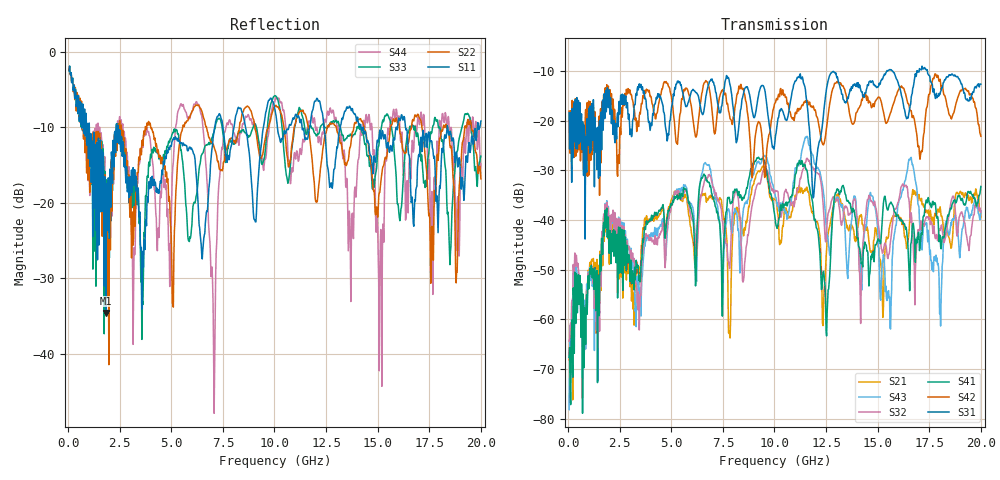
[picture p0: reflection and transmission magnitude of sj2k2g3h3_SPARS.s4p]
! FILE: E:\users\goganessyan\GBX_Backplane\FR408_backplane\1m_OUTBOUND_NEXT\sj2k2g3h3_SPARS.s4p
# MHZ S RI R 50.00
! FREQ  S11  S12  S13  S14
!  S21  S22  S23  S24
!  S31  S32  S33  S34
!  S41  S42  S43  S44
!  REAL  IMAG  REAL  IMAG  REAL  IMAG  REAL  IMAG
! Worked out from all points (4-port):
!   799 points, 50 MHz to 20 GHz, reference 50 ohm
!   strongest paths, dB at 50 MHz, 5.025 GHz, 10.03 GHz, 15.03 GHz, 20 GHz:
!     S31: -18.4, -17.0, -24.0, -13.2, -12.7
!     S42: -18.1, -15.9, -16.5, -15.3, -23.2
!     S41: -67.6, -37.0, -39.5, -43.8, -33.3
!     S32: -64.4, -36.7, -34.1, -40.9, -38.5
!     S43: -78.1, -36.9, -34.8, -44.3, -38.2
!     S21: -68.1, -35.7, -35.9, -45.4, -39.5
!   lowest |S11| = -34.6 dB at 1.825 GHz (marker M1), VSWR 1.04, Z = 51.7 + j0.726 ohm
!   |S11| at or under -10 dB: 2.428 GHz to 7.099 GHz (4.67 GHz wide, 98 % of centre); 14.3 GHz to 15.9 GHz (1.596 GHz wide, 10.6 % of centre); 16.35 GHz to 18.37 GHz (2.018 GHz wide, 11.6 % of centre)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
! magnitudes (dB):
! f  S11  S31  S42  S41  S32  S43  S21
! 50 MHz  -2.5  -18.4  -18.1  -67.6  -64.4  -78.1  -68.1
! 1.825 GHz  -34.6  -14.0  -17.9  -41.6  -40.5  -39.6  -42.4
! 7.075 GHz  -10.3  -12.9  -22.4  -36.3  -34.1  -34.6  -35.5
! 7.825 GHz  -13.8  -12.5  -19.1  -35.9  -49.8  -38.5  -62.9
! 11.28 GHz  -8.9  -11.5  -17.5  -28.8  -31.7  -27.6  -34.2
! 12.55 GHz  -14.9  -13.0  -20.5  -58.7  -40.5  -43.0  -44.4
! 20 GHz  -9.2  -12.7  -23.2  -33.3  -38.5  -38.2  -39.5
